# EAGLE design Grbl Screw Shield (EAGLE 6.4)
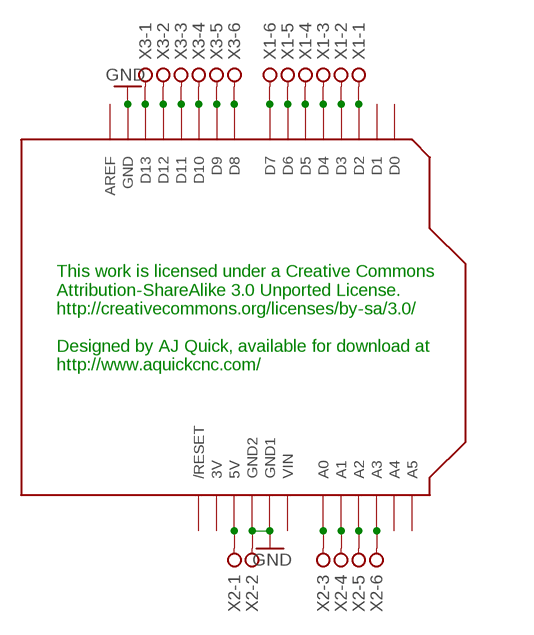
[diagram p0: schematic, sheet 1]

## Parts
U$1  ARDUINOUNO  [ARDUINO]
X1  W237-06P  [W237-6P]
X2  W237-06P  [W237-6P]
X3  W237-06P  [W237-6P]

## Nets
GND: U$1.GND U$1.GND1 U$1.GND2 X2.2
N$1: U$1.D7 X1.6
N$2: U$1.D6 X1.5
N$3: U$1.D4 X1.3
N$4: U$1.D5 X1.4
N$5: U$1.D3 X1.2
N$6: U$1.D2 X1.1
N$7: U$1.5V X2.1
N$8: U$1.D8 X3.6
N$9: U$1.A0 X2.3
N$10: U$1.A1 X2.4
N$11: U$1.A2 X2.5
N$12: U$1.A3 X2.6
N$13: U$1.D9 X3.5
N$14: U$1.D10 X3.4
N$15: U$1.D11 X3.3
N$16: U$1.D12 X3.2
N$17: U$1.D13 X3.1
Unconnected: U$1.A4 U$1.A5 U$1.AREF U$1.D0 U$1.D1 U$1.RESET(/RESET)

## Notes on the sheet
- This work is licensed under a Creative Commons
  Attribution-ShareAlike 3.0 Unported License.
  http://creativecommons.org/licenses/by-sa/3.0/
  
  Designed by AJ Quick, available for download at
  http://www.aquickcnc.com/

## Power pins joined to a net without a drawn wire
3V: U$1.3V
VIN: U$1.VIN

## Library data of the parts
U$1 = adafruit:ARDUINO: Arduino Diecimila/Duemilanove Make a shield with ease, this package has all the named pins as well as the two mounting drill holes and an outline of the USB and DC power connector. The outline is on the DIMENSION layer, so if your board house uses it they will cut the outline to match.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
X1-X3 = con-wago-508:W237-06P: WAGO SREW CLAMP; OC_FARNELL: unknown; OC_NEWARK: unknown

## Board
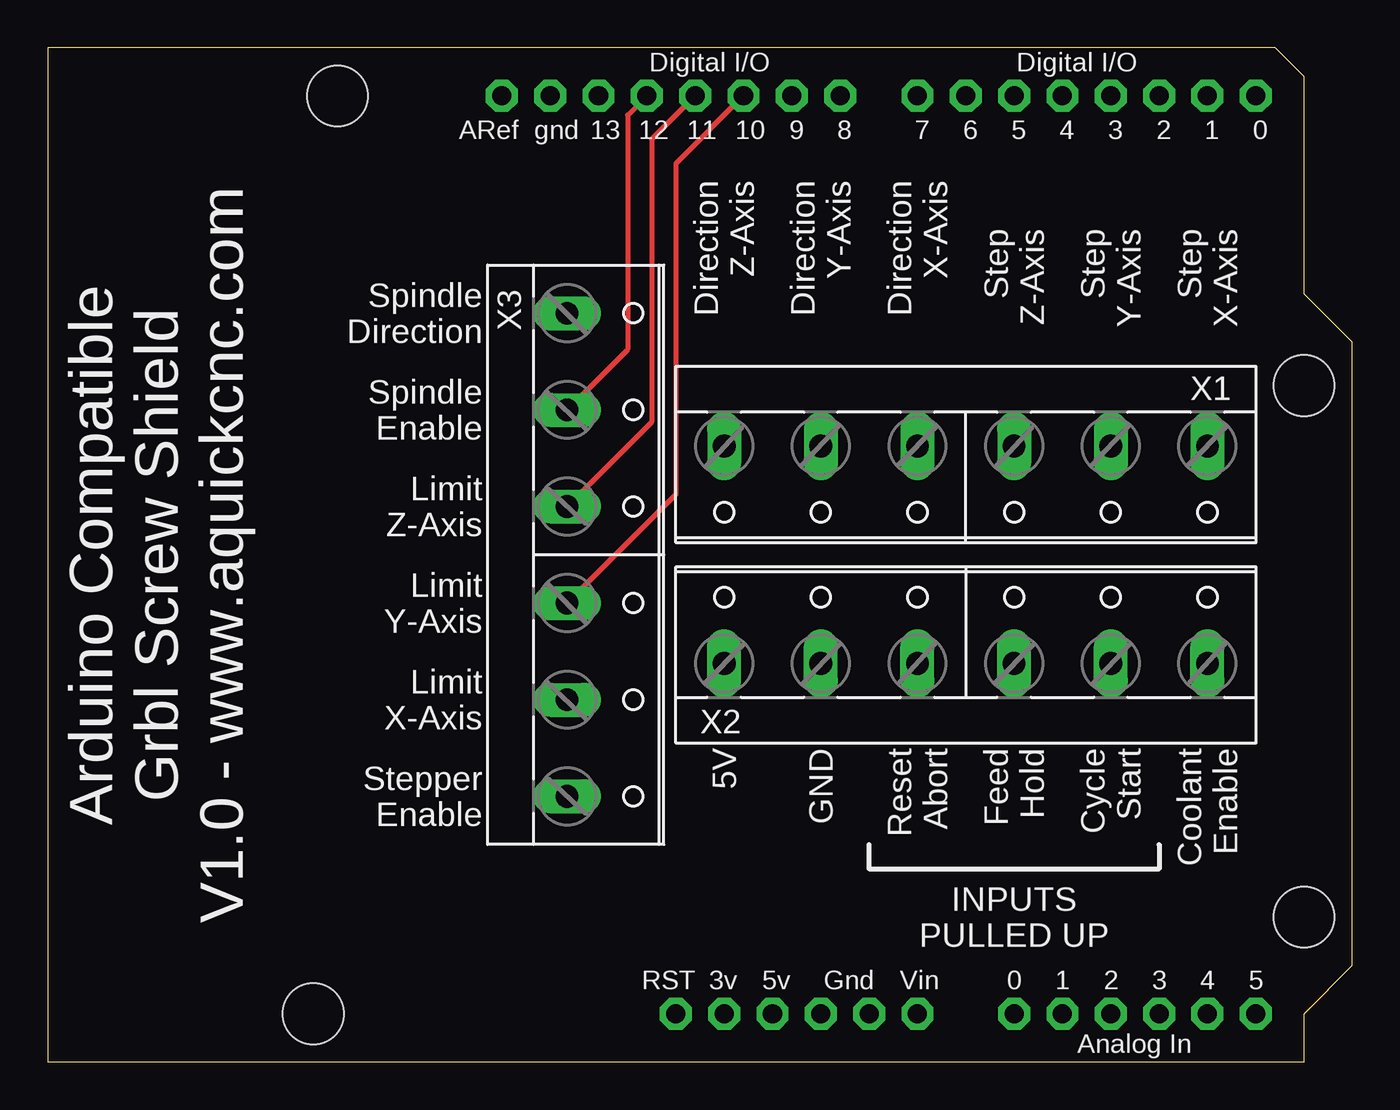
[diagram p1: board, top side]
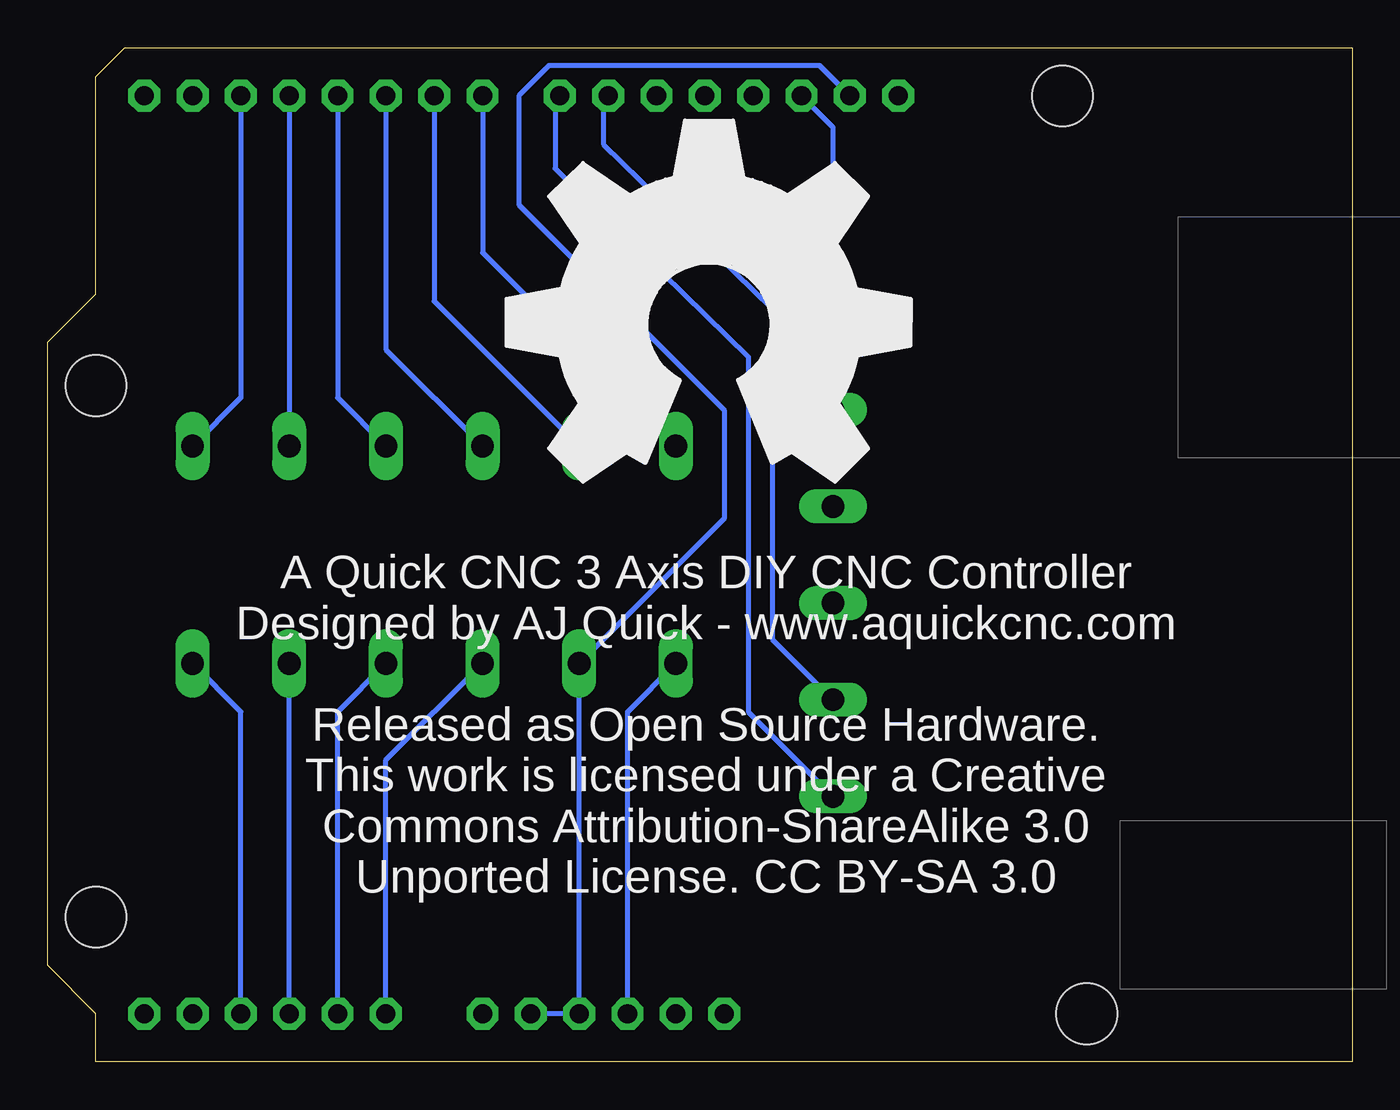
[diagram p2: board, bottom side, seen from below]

Size 68.58 x 53.34 mm. Coordinates in mm from the lower left corner, seen from the top.
Copper layers (1*2*15*16): Top 0.035mm / dielectric 0.2mm / Route2 0.0175mm / dielectric 1.1mm / Route15 0.0175mm / dielectric 0.2mm / Bottom 0.035mm
Design rules "SeeedStudio_DRU_no_angle_20130527": minimum track width 6mil, minimum drill 12mil, track to track 6mil, track to pad 6mil, pad to pad 6mil, via to via 6mil, smd to smd 0mil, copper to edge 10mil, drill to drill 10mil, minimum pad ring 6mil, minimum via ring 6mil, stop-mask expansion 2mil, vias tented up to drill 25mil, thermal gap 10mil

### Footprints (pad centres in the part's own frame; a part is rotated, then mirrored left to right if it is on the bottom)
ARDUINO = drill 1 pad 1.676 octagon: 3V 35.56,2.54; 5V 38.1,2.54; A0 50.8,2.54; A1 53.34,2.54; A2 55.88,2.54; A3 58.42,2.54; A4 60.96,2.54; A5 63.5,2.54; AREF 23.876,50.8; D0 63.5,50.8; D1 60.96,50.8; D2 58.42,50.8; D3 55.88,50.8; D4 53.34,50.8; D5 50.8,50.8; D6 48.26,50.8; D7 45.72,50.8; D8 41.656,50.8; D9 39.116,50.8; D10 36.576,50.8; D11 34.036,50.8; D12 31.496,50.8; D13 28.956,50.8; GND 26.416,50.8; GND1 43.18,2.54; GND2 40.64,2.54; RESET 33.02,2.54; VIN 45.72,2.54 | hole 3.2: 15.24,50.8; 66.04,35.56; 13.97,2.54; 66.04,7.62
W237-6P = drill 1.194 long: 1 -12.7,-0.635; 2 -7.62,-0.635; 3 -2.54,-0.635; 4 2.54,-0.635; 5 7.62,-0.635; 6 12.7,-0.635

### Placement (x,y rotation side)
U$1  0,0 0 top
U$2  [OSHW_FILLX750_NOTEXT]  44.45,30.48 0 bottom
X1  48.26,31.75 180 top
X2  48.26,21.59 0 top
X3  27.94,26.67 270 top

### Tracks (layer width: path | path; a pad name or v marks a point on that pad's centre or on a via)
GND
  Bottom 0.254: U$1.GND1 U$1.GND2 X2.2 33.02,28.57 33.02,34.29 43.81,45.09 43.81,50.8 42.23,52.39 28,52.39 U$1.GND
N$1
  Bottom 0.254: U$1.D7 45.72,42.55 X1.6
N$2
  Bottom 0.254: U$1.D6 48.26,40.01 X1.5
N$3
  Bottom 0.254: U$1.D4 53.34,34.92 X1.3
N$4
  Bottom 0.254: U$1.D5 50.8,37.47 X1.4
N$5
  Bottom 0.254: U$1.D3 X1.2
N$6
  Bottom 0.254: U$1.D2 58.42,34.92 X1.1
N$7
  Bottom 0.254: U$1.5V 38.1,18.41 X2.1
N$8
  Bottom 0.254: U$1.D8 41.91,50.8 41.91,46.99 31.75,37.08 31.75,18.41 X3.6
N$9
  Bottom 0.254: U$1.A0 50.8,15.88 X2.3
N$10
  Bottom 0.254: U$1.A1 53.34,18.41 X2.4
N$11
  Bottom 0.254: U$1.A2 X2.5
N$12
  Bottom 0.254: U$1.A3 58.42,18.41 X2.6
N$13
  Bottom 0.254: U$1.D9 39.37,50.8 39.37,48.26 30.48,39.62 30.48,22.23 X3.5
N$14
  Top 0.254: U$1.D10 33.02,47.24 33.02,29.84 X3.4
N$15
  Top 0.254: U$1.D11 31.75,48.51 31.75,33.66 X3.3
N$16
  Top 0.254: U$1.D12 30.48,49.78 30.48,37.47 X3.2
N$17
  Bottom 0.254: U$1.D13 27.3,49.15 X3.1

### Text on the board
bPlace: A Quick CNC 3 Axis DIY CNC Controller / Designed by AJ Quick - www.aquickcnc.com / / Released as Open Source Hardware. / This work is licensed under a Creative / Commons Attribution-ShareAlike 3.0 / Unported License. CC BY-SA 3.0
tNames: Direction / Z-Axis | Direction / Y-Axis | Direction / X-Axis | Step / Z-Axis | Step / Y-Axis | Step / X-Axis | Spindle / Direction | Spindle / Enable | Limit / Z-Axis | Arduino Compatible / Grbl Screw Shield / V1.0 - www.aquickcnc.com | Limit / Y-Axis | Limit / X-Axis | 5V | GND | Reset / Abort | Feed / Hold | Cycle / Start | Coolant / Enable | Stepper / Enable | INPUTS / PULLED UP
200bmp: Z:/My Documents/eagle/quickcnc-logo - Copy - Copy.bmp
